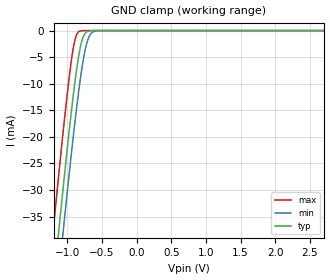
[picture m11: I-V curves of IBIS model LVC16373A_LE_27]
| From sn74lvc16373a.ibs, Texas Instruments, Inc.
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[Model]   LVC16373A_LE_27
Model_type  Input
Vinl = 0.7
Vinh = 1.7
| variable   typ   min   max
C_comp   4.44pF   3.65pF   5.41pF
[Temperature Range]   40   100   -40
| Ambient temperature   25   85   -40
[Voltage range]   2.7   2.7   2.7
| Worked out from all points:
|   GND clamp passes 1 mA (typ) near -0.77 V on its own axis
[GND Clamp]
| LVC16373A_LE_27
|   Voltage   I(typ)   I(min)   I(max)
-5.5V     -655.9mA   -662.8mA   -647.2mA
-1.205V   -48.32mA   -56.61mA   -37.67mA
-1.13V    -38.46mA   -46.75mA   -27.8mA
-1.07V    -30.74mA   -39mA      -20.15mA
-1.055V   -28.84mA   -37.09mA   -18.29mA
-955mV    -16.69mA   -24.69mA   -6.88mA
-885mV    -9.107mA   -16.56mA   -1.487mA
-825mV    -3.926mA   -10.27mA   -137.3uA
-780mV    -1.473mA   -6.233mA   -17.16uA
-715mV    -205.6uA   -2.13mA    -809.3nA
-645mV    -18.5uA    -388uA     -30.01nA
2.7V      5.111pA    7.76pA     4.886pA
